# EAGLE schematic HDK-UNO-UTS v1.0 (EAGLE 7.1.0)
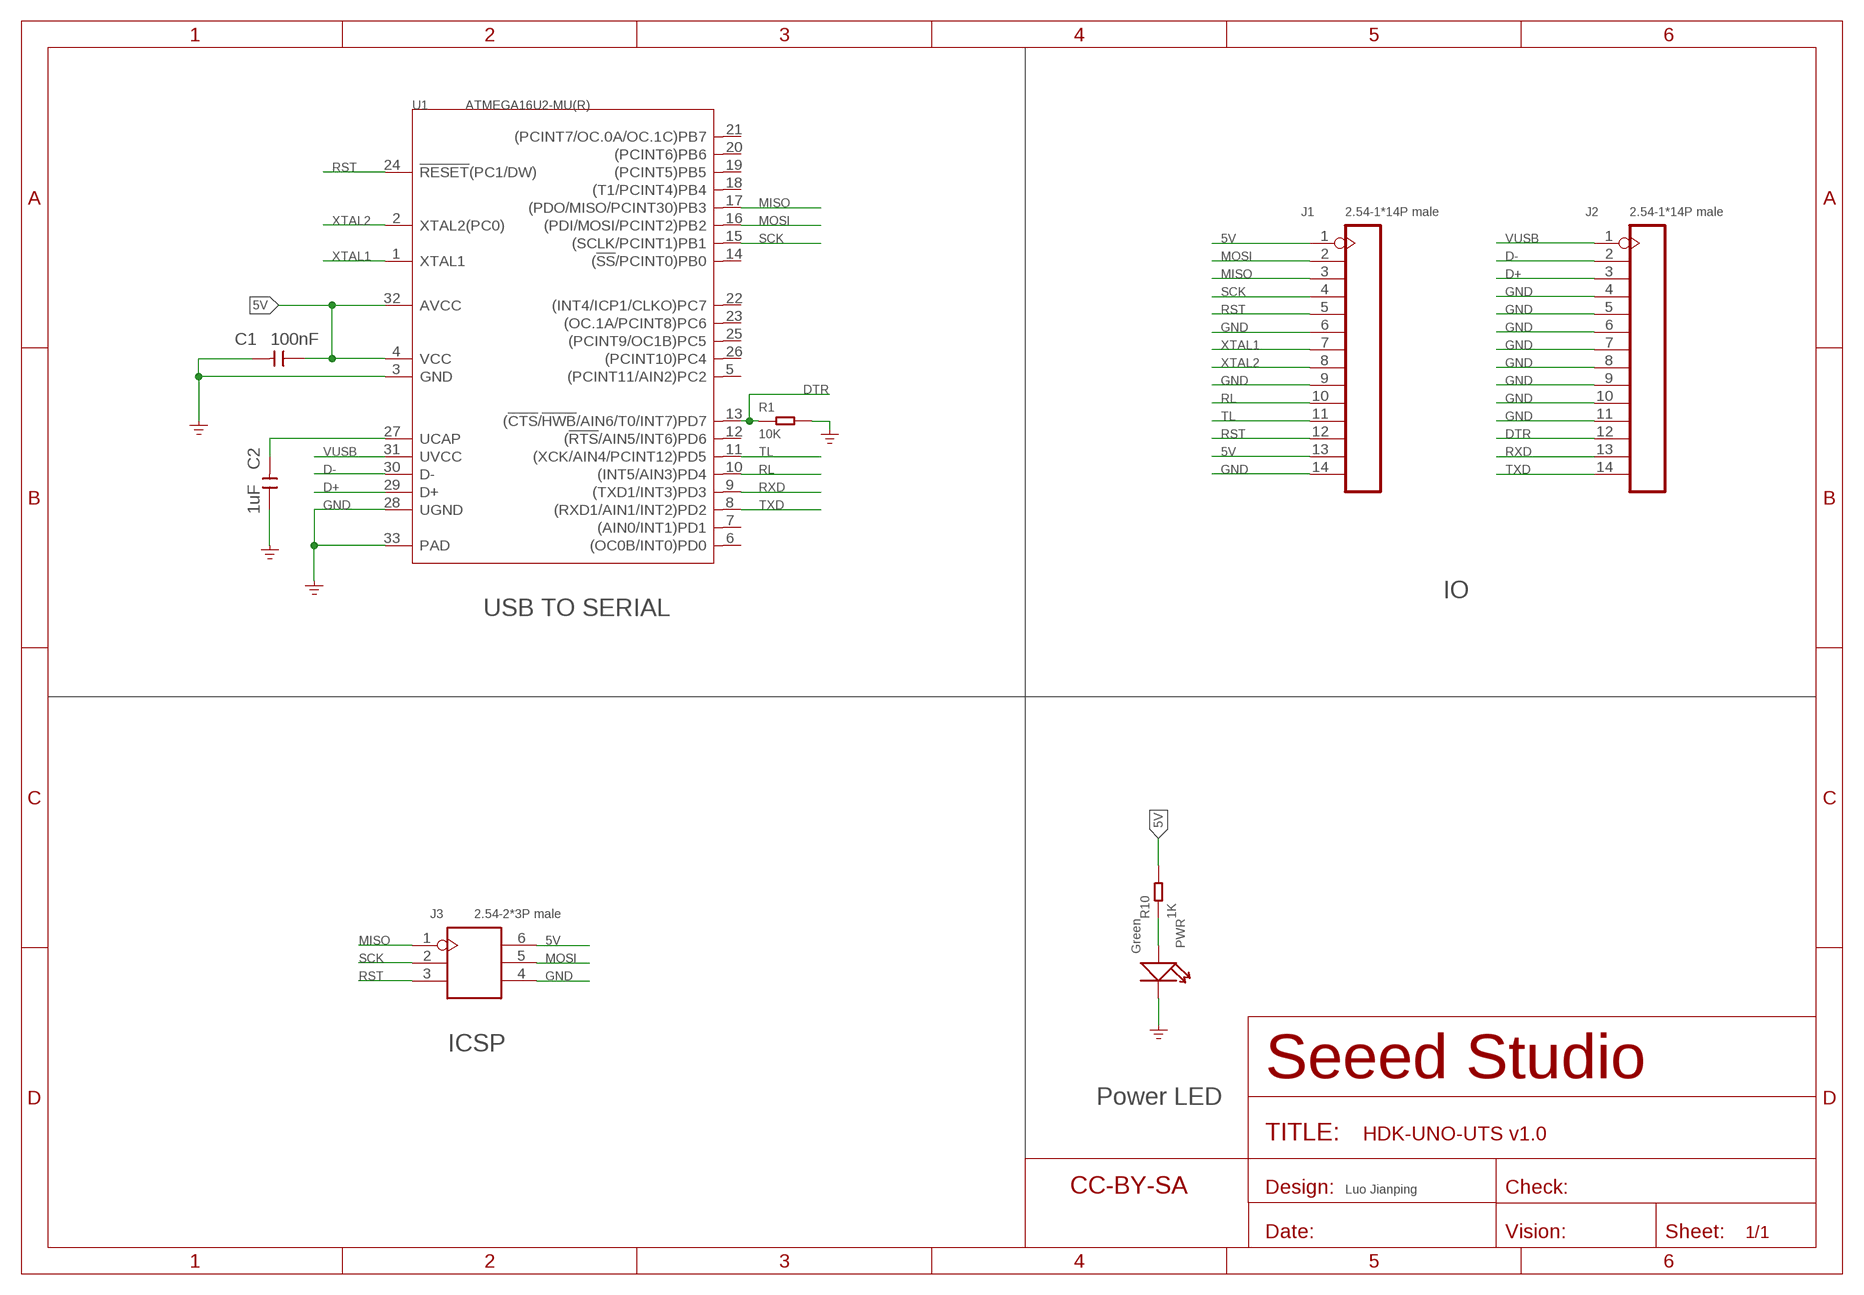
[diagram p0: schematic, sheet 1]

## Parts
C1  100nF  CAP-0603  [C0603]
C2  1uF  CAP-0603  [C0603]
FR  SEEEDSTUDIO-OPEN-SCH-FRAME  [SEEEDSTUDIO-PCB-FRAME]
J1  2.54-1*14P male  HEADER-14P-2.54  [H14-2.54]
J2  2.54-1*14P male  HEADER-14P-2.54  [H14-2.54]
J3  2.54-2*3P male  HEADER-2X3P-2.54  [H2X3-2.54]
PWR  Green  LED'0603'  [LED-0603]
R1  10K  RES-0603  [R0603]
R10  1K  RES-0603  [R0603]
U1  ATMEGA16U2-MU(R)  CONTROLLER-ATMEGA16U2  [QFN32G-0.5-5X5MM]

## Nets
5V: C1.1 J1.1 J1.13 J3.6 R10.2 U1.4(VCC) U1.32(AVCC)
D+: J2.3 U1.29(D+)
D-: J2.2 U1.30(D-)
DTR: J2.12 R1.1 U1.13((!CTS!/!HWB!/AIN6/T0/INT7)PD7)
GND [none1]: C1.2 C2.1 J1.6 J1.9 J1.14 J2.4 J2.5 J2.6 J2.7 J2.8 J2.9 J2.10 J2.11 J3.4 PWR.- R1.2 U1.3(GND) U1.28(UGND) U1.33(PAD) ; supply symbol labelled GND_POWER
MISO: J1.3 J3.1 U1.17((PDO/MISO/PCINT30)PB3)
MOSI: J1.2 J3.5 U1.16((PDI/MOSI/PCINT2)PB2)
N$3: PWR.+ R10.1
N$9: C2.2 U1.27(UCAP)
RL: J1.10 U1.10((INT5/AIN3)PD4)
RST: J1.5 J1.12 J3.3 U1.24(!RESET!(PC1/DW))
RXD: J2.13 U1.9((TXD1/INT3)PD3)
SCK: J1.4 J3.2 U1.15((SCLK/PCINT1)PB1)
TL: J1.11 U1.11((XCK/AIN4/PCINT12)PD5)
TXD: J2.14 U1.8((RXD1/AIN1/INT2)PD2)
VUSB: J2.1 U1.31(UVCC)
XTAL1: J1.7 U1.1(XTAL1)
XTAL2: J1.8 U1.2(XTAL2(PC0))
Unconnected: U1.5((PCINT11/AIN2)PC2) U1.6((OC0B/INT0)PD0) U1.7((AIN0/INT1)PD1) U1.12((!RTS!/AIN5/INT6)PD6) U1.14((!SS!/PCINT0)PB0) U1.18((T1/PCINT4)PB4) U1.19((PCINT5)PB5) U1.20((PCINT6)PB6) U1.21((PCINT7/OC.0A/OC.1C)PB7) U1.22((INT4/ICP1/CLKO)PC7) U1.23((OC.1A/PCINT8)PC6) U1.25((PCINT9/OC1B)PC5) U1.26((PCINT10)PC4)

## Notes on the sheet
- IO
- USB TO SERIAL
- ICSP
- Power LED
- Luo Jianping

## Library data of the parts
C1 C2 = Discrete-new:CAP: Ceramic Capacitors
FR = moudle-new:SEEEDSTUDIO-OPEN-SCH-FRAME
J1 J2 = Connector-new:HEADER-14P: Header 14 Standard 14-pin 0.1" header. Use with straight break away headers (SKU : PRT-00116), right angle break away headers (PRT-00553), swiss pins (PRT-00743), machine pins (PRT-00117), and female headers (PRT-00115).
J3 = Connector-new:HEADER-2X3P
PWR = Discrete-new:LED
R1 R10 = Discrete-new:RES
U1 = IC-new:CONTROLLER-ATMEGA16U2: 310010018

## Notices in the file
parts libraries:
moudle-new: This work is licensed under the Creative Commons Attribution 4.0 International License.
To view a copy of this license,visit:
http://creativecommons.org/licenses/by-sa/4.0
moudle-new: CC-BY-SA
